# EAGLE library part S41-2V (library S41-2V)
General Purpose Relays,Wide switching range From 100A 100 mV DC to 4 A 250 V AC Source: Datasheet
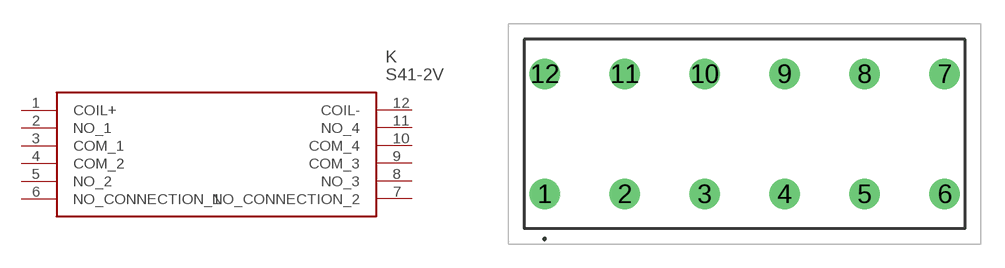
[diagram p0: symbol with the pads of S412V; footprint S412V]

Designator prefix K

## S41-2V (Description: General Purpose Relays,Wide switching range From 100A 100 mV DC to 4 A 250 V AC; Height: 10.9mm; Manufacturer_Name: Panasonic; Manufacturer_Part_Number: S41-2V)  [S412V]
1  COIL+
2  NO_1
3  COM_1
4  COM_2
5  NO_2
6  NO_CONNECTION_1
7  NO_CONNECTION_2
8  NO_3
9  COM_3
10  COM_4
11  NO_4
12  COIL-

## Footprint S412V (pad centres in mm)
S412V-3
drill 1.3 pad 1.95: 1 0,0; 2 5.08,0; 3 10.16,0; 4 15.24,0; 5 20.32,0; 6 25.4,0; 7 25.4,7.62; 8 20.32,7.62; 9 15.24,7.62; 10 10.16,7.62; 11 5.08,7.62; 12 0,7.62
